| IBIS file generated by GenIBIS.exe Version 3.25
|   am335x_zcz
[IBIS ver]   4.1
[File name]   sprm552c.ibs
[File Rev]   1.1
[Date]   02/05/2016
[Source]   Data created at Texas Instruments
[Notes]   1) Checked with IBISCHK5.0.0 with the following exceptions...
   417 warnings. These warnings can be waived.
   2) Model not valid until this section updated.
   Some pins may contain selectors which are not valid options
   for that particular pin.
   Please refer to the device datasheet for information on picking
   the correct selector model, which depends on various software
   register configurations.
   Some pins are modeled as IO or tri-state for output mode.
[Disclaimer] Please be aware that in the absence of a written agreement,
   Texas Instruments (TI) assumes no liability for: 1) the
   accuracy of the IBIS models provided to your company, 2) the
   proper functioning of these IBIS models in your design or for
   any resulting applications, or, 3) infringement of patents,
   copyrights, or intellectual property rights resulting from
   your use of these IBIS models. TI provides IBIS models as a
   service to our customers and therefore reserves the right to
   limit distribution of the IBIS models.
[Copyright]   Property of Texas Instruments Incorporated. Unauthorised
   reproduction and/or distribution is strictly prohibited. This
   product is protected under copyright law and trade secret law
   as an unpublished work. Created 2016,(C) Copyright 2010,
   Texas Instruments Incorporated., All Rights Reserved. These
   commodities are under the U.S. Government distribution license
   control.As such,they are not to be re-exported without the
   prior approval of the U.S. Department of Commerce.
|   Component am335x_zcz
[Component]   am335x_zce
[Manufacturer]   Texas Instruments.
| Source IO level model revisions
|Model   Revision   Date
|BC1833DV40DCPBFBP18LL_SSDHH   1.1   May 27, 2010
|BC1833DV50BPBFBP18LL_SSDLV   1.0   May 30, 2010
|BC1833DV50BPBFBP18LL_SSDHV   1.1   May 30, 2010
|OQ18SMART1FBPB_SSBHH   1.0   Dec 17, 2008
|BC1833DV40DCPBFBP18LL_SSDLV   1.0   May 27, 2010
|IQ18HYENPB_SSBHH   1.0   May 2, 2008
|BC1833DV50BPBFBP18LL_SSDLH   1.0   May 30, 2010
|BC1833DV40DCPBFBP18LL_SSDHV   1.1   May 27, 2010
|IQ1833DVTCKPBFBP18LL_SSDHH   1.1   May 27, 2010
|IQ18GLFHY_SSBHH   1.0   May 2, 2008
|IHHV1833DVHYP18LL_SSDHH   1.1   May 27, 2010
|BC1833DV50BPBFBP18LL_SSDHH   1.1   May 30, 2010
|BC1833DV40DCPBFBP18LL_SSDLH   1.0   May 27, 2010
|IC1833DVPBFBP18LL_SSDHH   1.1   May 27, 2010
|BCSHTLTCSCDVPBFZ_SSDHV   1.0   May 31, 2010
|BCSHTLTCSCDDVPBFZ_SSDHV   1.0   May 31, 2010
[Package Model] am335x_zce
[Package]
|   typ   min   max
R_pkg   0.22666002591133e-  1.48102e-03   4.40563e-01
L_pkg   3.34766526650246E-009e- 3.63859e-11   7.90050e-09
C_pkg   1.03822401477832E-012e- 3.34415e-13   3.16645e-11
[Pin]   signal_name   model_name
B8   AIN0   NC
A11   AIN1   NC
A8   AIN2   NC
B11   AIN3   NC
C8   AIN4   NC
B12   AIN5   NC
A10   AIN6   NC
A12   AIN7   NC
C13   CAP_VBB_MPU   NC
D6   CAP_VDD_RTC   POWER
B10   CAP_VDD_SRAM_CORE   NC
D13   CAP_VDD_SRAM_MPU   NC
N3   DDR_DQM0   Selector_4
F3   DDR_A0   Selector_4
J1   DDR_VTP   NC
B4   DDR_BA2   Selector_4
H3   DDR_A14   Selector_4
M4   DDR_D11   Selector_11
D2   DDR_A7   Selector_4
G3   DDR_CKE   Selector_4
A3   DDR_BA0   Selector_4
F2   DDR_RASN   Selector_4
P3   DDR_D4   Selector_11
M1   DDR_D13   Selector_11
L1   DDR_DQS1   Selector_1
P1   DDR_D3   Selector_11
F4   DDR_A12   Selector_4
N1   DDR_D15   Selector_11
K2   DDR_D8   Selector_11
R1   DDR_DQS0   Selector_1
L2   DDR_DQSN1   Selector_6
E5   DDR_A4   Selector_4
J2   DDR_A1   Selector_4
G1   DDR_ODT   Selector_4
T1   DDR_D5   Selector_11
A4   DDR_WEN   Selector_4
G4   DDR_A11   Selector_4
E2   DDR_A10   Selector_4
B3   DDR_A3   Selector_4
H2   DDR_CSN0   Selector_4
E3   DDR_A15   Selector_4
G2   DDR_RESETN   Selector_4
C2   DDR_CK   Selector_4
P2   DDR_D2   Selector_11
F1   DDR_CASN   Selector_4
R3   DDR_D7   Selector_11
K3   DDR_DQM1   Selector_4
K1   DDR_D9   Selector_11
A2   DDR_A5   Selector_4
N4   DDR_D0   Selector_11
B2   DDR_A9   Selector_4
M2   DDR_D12   Selector_11
H4   DDR_VREF   NC
N2   DDR_D14   Selector_11
D1   DDR_A2   Selector_4
M3   DDR_D10   Selector_11
R2   DDR_DQSN0   Selector_6
C1   DDR_CKN   Selector_4
T2   DDR_D6   Selector_11
E1   DDR_BA1   Selector_4
H1   DDR_A13   Selector_4
B1   DDR_A6   Selector_4
P4   DDR_D1   Selector_11
C3   DDR_A8   Selector_4
E18   ECAP0_IN_PWM0_OUT   Selector_12
A15   EMU0   Selector_14
D14   EMU1   Selector_14
B5   EXT_WAKEUP   Selector_5
C17   EXTINTN   Selector_7
V17   GPMC_AD15   Selector_15
V15   GPMC_AD8   Selector_15
V12   GPMC_AD2   Selector_15
V10   GPMC_ADVN_ALE   Selector_14
R15   GPMC_WAIT0   Selector_14
U13   GPMC_AD12   Selector_15
T13   GPMC_AD13   Selector_15
U12   GPMC_AD11   Selector_15
V14   GPMC_CSN1   Selector_15
W14   GPMC_AD5   Selector_15
W13   GPMC_AD3   Selector_15
U17   GPMC_CSN3   Selector_15
W8   GPMC_CSN0   Selector_14
T12   GPMC_AD10   Selector_15
U15   GPMC_CSN2   Selector_15
W18   GPMC_WPN   Selector_15
V9   GPMC_AD1   Selector_15
W9   GPMC_OEN_REN   Selector_14
V8   GPMC_BEN0_CLE   Selector_14
W16   GPMC_AD9   Selector_15
V18   GPMC_BEN1   Selector_15
V13   GPMC_AD4   Selector_15
W15   GPMC_AD7   Selector_15
U14   GPMC_AD6   Selector_15
W17   GPMC_AD14   Selector_15
V16   GPMC_CLK   Selector_15
U8   GPMC_WEN   Selector_14
W10   GPMC_AD0   Selector_14
C18   I2C0_SDA   Selector_16
B19   I2C0_SCL   Selector_16
W2   LCD_DATA4   Selector_17
V5   LCD_DATA11   Selector_10
W5   LCD_PCLK   Selector_10
V3   LCD_DATA6   Selector_17
W7   LCD_AC_BIAS_EN   Selector_14
U1   LCD_DATA0   Selector_17
U5   LCD_DATA10   Selector_10
U7   LCD_VSYNC   Selector_14
V2   LCD_DATA3   Selector_17
W3   LCD_DATA5   Selector_17
U6   LCD_DATA13   Selector_17
W4   LCD_DATA9   Selector_10
V7   LCD_DATA15   Selector_14
V6   LCD_DATA12   Selector_17
U3   LCD_DATA7   Selector_10
V1   LCD_DATA2   Selector_17
V4   LCD_DATA8   Selector_10
W6   LCD_DATA14   Selector_15
T7   LCD_HSYNC   Selector_14
U2   LCD_DATA1   Selector_17
R19   MDC   Selector_10
P17   MDIO   Selector_10
L18   MII1_TXD0   Selector_10
J18   MII1_CRS   Selector_10
N18   MII1_TXD2   Selector_10
J19   MII1_COL   Selector_10
N19   MII1_TX_CLK   Selector_10
M17   MII1_TXD3   Selector_10
M18   MII1_TXD1   Selector_10
N16   MII1_RXD2   Selector_10
M19   MII1_RX_CLK   Selector_10
P18   MII1_RXD0   Selector_10
K19   MII1_RX_ER   Selector_10
K17   MII1_TX_EN   Selector_10
P19   MII1_RXD1   Selector_10
N17   MII1_RXD3   Selector_10
L19   MII1_RX_DV   Selector_10
G17   MMC0_CMD   Selector_10
H17   MMC0_DAT1   Selector_10
H18   MMC0_DAT2   Selector_10
G19   MMC0_CLK   Selector_10
G18   MMC0_DAT0   Selector_10
H19   MMC0_DAT3   Selector_10
C7   PMIC_POWER_EN   Selector_2
E15   PWRONRSTN   Selector_3
B6   RESERVED   NC
K18   RMII1_REF_CLK   Selector_10
B7   RTC_PWRONRSTN   Model_172
A6   RTC_XTALIN   NC
A5   RTC_XTALOUT   NC
A7   RTC_KALDO_ENN   NC
A18   SPI0_SCLK   Selector_14
B16   SPI0_CS1   Selector_14
B18   SPI0_D0   Selector_14
A17   SPI0_CS0   Selector_14
B17   SPI0_D1   Selector_14
B14   TCK   Selector_8
B13   TDI   Selector_19
A14   TDO   Selector_13
C14   TMS   Selector_18
A13   TRSTN   Selector_19
E19   UART0_RXD   Selector_12
F17   UART0_TXD   Selector_12
F18   UART0_RTSN   Selector_12
F19   UART0_CTSN   Selector_12
D18   UART1_RXD   Selector_12
D19   UART1_RTSN   Selector_12
C19   UART1_TXD   Selector_12
E17   UART1_CTSN   Selector_12
T18   USB0_CE   NC
U18   USB0_DM   NC
T19   USB0_VBUS   NC
V19   USB0_ID   NC
G16   USB0_DRVVBUS   Selector_12
U19   USB0_DP   NC
F11   VDD_CORE   POWER
F9   VDD_CORE   POWER
G11   VDD_CORE   POWER
G9   VDD_CORE   POWER
H12   VDD_CORE   POWER
H13   VDD_CORE   POWER
H7   VDD_CORE   POWER
H8   VDD_CORE   POWER
J12   VDD_CORE   POWER
J13   VDD_CORE   POWER
J7   VDD_CORE   POWER
J8   VDD_CORE   POWER
K15   VDD_CORE   POWER
K16   VDD_CORE   POWER
L12   VDD_CORE   POWER
L13   VDD_CORE   POWER
L7   VDD_CORE   POWER
L8   VDD_CORE   POWER
M12   VDD_CORE   POWER
M13   VDD_CORE   POWER
M7   VDD_CORE   POWER
M8   VDD_CORE   POWER
N11   VDD_CORE   POWER
N9   VDD_CORE   POWER
P11   VDD_CORE   POWER
P9   VDD_CORE   POWER
D7   VDDA_ADC   POWER
R17   VDDA1P8V_USB0   POWER
R18   VDDA3P3V_USB0   POWER
G5   VDDS_DDR   POWER
H5   VDDS_DDR   POWER
H6   VDDS_DDR   POWER
K4   VDDS_DDR   POWER
K5   VDDS_DDR   POWER
M5   VDDS_DDR   POWER
M6   VDDS_DDR   POWER
N5   VDDS_DDR   POWER
U10   VDDS_OSC   POWER
C6   VDDS_RTC   POWER
C5   VDDS_PLL_DDR   POWER
D12   VDDS   POWER
F16   VDDS   POWER
M16   VDDS   POWER
T14   VDDS   POWER
T6   VDDS   POWER
T8   VDDS_PLL_CORE_LCD   POWER
C12   VDDS_SRAM_MPU_BB   POWER
H16   VDDS_PLL_MPU   POWER
C10   VDDS_SRAM_CORE_BG   POWER
R11   VDDSHV1   POWER
R12   VDDSHV1   POWER
R13   VDDSHV1   POWER
R8   VDDSHV1   POWER
R9   VDDSHV1   POWER
G15   VDDSHV4   POWER
H14   VDDSHV4   POWER
H15   VDDSHV4   POWER
M14   VDDSHV5   POWER
M15   VDDSHV5   POWER
N15   VDDSHV5   POWER
E11   VDDSHV6   POWER
E12   VDDSHV6   POWER
E13   VDDSHV6   POWER
F14   VDDSHV6   POWER
P6   VDDSHV6   POWER
R7   VDDSHV6   POWER
R5   VPP   POWER
B9   VREFN   NC
A9   VREFP   NC
V11   VSS_OSC   GND
A1   VSS   GND
A19   VSS   GND
D10   VSS   GND
E10   VSS   GND
E7   VSS   GND
E8   VSS   GND
E9   VSS   GND
F12   VSS   GND
F13   VSS   GND
F6   VSS   GND
F7   VSS   GND
F8   VSS   GND
G12   VSS   GND
G8   VSS   GND
H10   VSS   GND
H11   VSS   GND
H9   VSS   GND
J11   VSS   GND
J14   VSS   GND
J15   VSS   GND
J5   VSS   GND
J6   VSS   GND
J9   VSS   GND
K11   VSS   GND
K12   VSS   GND
K8   VSS   GND
K9   VSS   GND
L11   VSS   GND
L14   VSS   GND
L15   VSS   GND
L5   VSS   GND
L6   VSS   GND
L9   VSS   GND
M10   VSS   GND
M11   VSS   GND
M9   VSS   GND
N12   VSS   GND
N8   VSS   GND
P12   VSS   GND
P13   VSS   GND
P14   VSS   GND
P7   VSS   GND
P8   VSS   GND
R10   VSS   GND
T10   VSS   GND
W1   VSS   GND
W19   VSS   GND
P16   VSSA_USB   GND
D8   VSSA_ADC   GND
A16   WARMRSTN   Selector_9
C15   XDMA_EVENT_INTR0   Selector_16
B15   XDMA_EVENT_INTR1   Selector_16
W11   XTALIN   NC
W12   XTALOUT   NC
[Diff Pin] inv_pin  vdiff  tdelay_typ
|Differential signal data for cell BCSHTLTCSCDDVPBFZ_SSDHV
|DDR_DQS1   DDR_DQSN1
L1   L2   200m   NA
|DDR_DQS0   DDR_DQSN0
R1   R2   200m   NA
|   Usage INPUT#1.35/1.5V/1.8V#X#X#BCSHTLTCSCDDVPBFZ_SSDHV.PADP
|   OUTPUT#1.35/1.5V/1.8V#X#X#BCSHTLTCSCDDVPBFZ_SSDHV.TX_P
|   Base model BCSHTLTCSCDDVPBFZ_SSDHV
[Model Selector] Selector_1
Model_1000 INPUT,1.5V,FULLTERM, 1.00*RExt,IND,5%,DIFF_VREF_FULLTERM_8MA_5PER_1P5
Model_1001 INPUT,1.5V,Half Thevenin, 1.60*RExt,IND,5%,DIFF_VREF_HALFTERM_5MA_5PER
Model_1002 INPUT,1.5V,FULLTERM, 0.88*RExt,IND,5%,DIFF_VREF_FULLTERM_9MA_5PER_1P5
Model_1003 INPUT,1.35V,Half Thevenin, 0.67*RExt,IND,10%,DIFF_VREF_HALFTERM_12MA_1
Model_1004 INPUT,1.35V,Pull-up/down off,IND,10%,DIFF_VREF_NOTERM_PUPD_OFF_10PER_1
Model_1005 INPUT,1.35V,FULLTERM, 1.60*RExt,IND,10%,DIFF_VREF_FULLTERM_5MA_10PER_1
Model_1006 INPUT,1.35V,Half Thevenin, 1.60*RExt,IND,10%,DIFF_VREF_HALFTERM_5MA_10
Model_1007 INPUT,1.35V,Pull-up,IND,10%,DIFF_VREF_NOTERM_PU_ON_10PER_1P35
Model_1008 INPUT,1.35V,FULLTERM, 0.88*RExt,IND,10%,DIFF_VREF_FULLTERM_9MA_10PER_1
Model_1009 INPUT,1.35V,FULLTERM, 1.14*RExt,IND,10%,DIFF_VREF_FULLTERM_7MA_10PER_1
Model_1010 INPUT,1.35V,Half Thevenin, 0.88*RExt,IND,10%,DIFF_VREF_HALFTERM_9MA_10
Model_1011 INPUT,1.35V,FULLTERM, 1.33*RExt,IND,10%,DIFF_VREF_FULLTERM_6MA_10PER_1
Model_1012 INPUT,1.35V,Half Thevenin, 1.14*RExt,IND,10%,DIFF_VREF_HALFTERM_7MA_10
Model_1013 INPUT,1.35V,Half Thevenin, 1.33*RExt,IND,10%,DIFF_VREF_HALFTERM_6MA_10
Model_1014 INPUT,1.35V,FULLTERM, 0.73*RExt,IND,10%,DIFF_VREF_FULLTERM_11MA_10PER_
Model_1015 INPUT,1.35V,FULLTERM, 0.80*RExt,IND,10%,DIFF_VREF_FULLTERM_10MA_10PER_
Model_1016 INPUT,1.35V,Half Thevenin, 0.73*RExt,IND,10%,DIFF_VREF_HALFTERM_11MA_1
Model_1017 INPUT,1.35V,FULLTERM, 1.00*RExt,IND,10%,DIFF_VREF_FULLTERM_8MA_10PER_1
Model_1018 INPUT,1.35V,Half Thevenin, 0.80*RExt,IND,10%,DIFF_VREF_HALFTERM_10MA_1
Model_1019 INPUT,1.35V,Pull-down,IND,10%,DIFF_VREF_NOTERM_PD_ON_10PER_1P35
Model_1020 INPUT,1.35V,Half Thevenin, 1.00*RExt,IND,10%,DIFF_VREF_HALFTERM_8MA_10
Model_1021 INPUT,1.35V,FULLTERM, 0.67*RExt,IND,10%,DIFF_VREF_FULLTERM_12MA_10PER_
Model_1022 INPUT,1.35V,Half Thevenin, 0.67*RExt,IND,5%,DIFF_VREF_HALFTERM_12MA_5P
Model_1023 INPUT,1.35V,Pull-up/down off,IND,5%,DIFF_VREF_NOTERM_PUPD_OFF_5PER_1P3
Model_1024 INPUT,1.35V,FULLTERM, 1.60*RExt,IND,5%,DIFF_VREF_FULLTERM_5MA_5PER_1P3
Model_1025 INPUT,1.35V,Half Thevenin, 1.60*RExt,IND,5%,DIFF_VREF_HALFTERM_5MA_5PE
Model_1026 INPUT,1.35V,Pull-up,IND,5%,DIFF_VREF_NOTERM_PU_ON_5PER_1P35
Model_1027 INPUT,1.35V,FULLTERM, 0.88*RExt,IND,5%,DIFF_VREF_FULLTERM_9MA_5PER_1P3
Model_1028 INPUT,1.35V,FULLTERM, 1.14*RExt,IND,5%,DIFF_VREF_FULLTERM_7MA_5PER_1P3
Model_1029 INPUT,1.35V,Half Thevenin, 0.88*RExt,IND,5%,DIFF_VREF_HALFTERM_9MA_5PE
Model_1030 INPUT,1.35V,FULLTERM, 1.33*RExt,IND,5%,DIFF_VREF_FULLTERM_6MA_5PER_1P3
Model_1031 INPUT,1.35V,Half Thevenin, 1.14*RExt,IND,5%,DIFF_VREF_HALFTERM_7MA_5PE
Model_1032 INPUT,1.35V,Half Thevenin, 1.33*RExt,IND,5%,DIFF_VREF_HALFTERM_6MA_5PE
Model_1033 INPUT,1.35V,FULLTERM, 0.73*RExt,IND,5%,DIFF_VREF_FULLTERM_11MA_5PER_1P
Model_1034 INPUT,1.35V,FULLTERM, 0.80*RExt,IND,5%,DIFF_VREF_FULLTERM_10MA_5PER_1P
Model_1035 INPUT,1.35V,Half Thevenin, 0.73*RExt,IND,5%,DIFF_VREF_HALFTERM_11MA_5P
Model_1036 INPUT,1.35V,FULLTERM, 1.00*RExt,IND,5%,DIFF_VREF_FULLTERM_8MA_5PER_1P3
Model_1037 INPUT,1.35V,Half Thevenin, 0.80*RExt,IND,5%,DIFF_VREF_HALFTERM_10MA_5P
Model_1038 INPUT,1.35V,Pull-down,IND,5%,DIFF_VREF_NOTERM_PD_ON_5PER_1P35
Model_1039 INPUT,1.35V,Half Thevenin, 1.00*RExt,IND,5%,DIFF_VREF_HALFTERM_8MA_5PE
Model_1040 INPUT,1.35V,FULLTERM, 0.67*RExt,IND,5%,DIFF_VREF_FULLTERM_12MA_5PER_1P
Model_537 3-STATE,1.8V,ODT off,slowest, 1.00*RExt,IND,10%,SR11_8MA_PADP_10PER_1P
Model_538 3-STATE,1.8V,ODT off,slowest, 1.60*RExt,IND,10%,SR11_5MA_PADP_10PER_1P
Model_539 3-STATE,1.8V,ODT off,fast, 1.14*RExt,IND,10%,SR10_7MA_PADP_10PER_1P8
Model_540 3-STATE,1.8V,ODT off,fast, 1.33*RExt,IND,10%,SR10_6MA_PADP_10PER_1P8
Model_541 3-STATE,1.8V,ODT off,slowest, 0.88*RExt,IND,10%,SR11_9MA_PADP_10PER_1P
Model_542 3-STATE,1.8V,ODT off,fast, 0.73*RExt,IND,10%,SR10_11MA_PADP_10PER_1P8
Model_543 3-STATE,1.8V,ODT off,slowest, 0.67*RExt,IND,10%,SR11_12MA_PADP_10PER_1
Model_544 3-STATE,1.8V,ODT off,slowest, 1.14*RExt,IND,10%,SR11_7MA_PADP_10PER_1P
Model_545 3-STATE,1.8V,ODT off,fast, 0.80*RExt,IND,10%,SR10_10MA_PADP_10PER_1P8
Model_546 3-STATE,1.8V,ODT off,slowest, 1.33*RExt,IND,10%,SR11_6MA_PADP_10PER_1P
Model_547 3-STATE,1.8V,ODT off,fast, 1.00*RExt,IND,10%,SR10_8MA_PADP_10PER_1P8
Model_548 3-STATE,1.8V,ODT off,fast, 1.60*RExt,IND,10%,SR10_5MA_PADP_10PER_1P8
Model_549 3-STATE,1.8V,ODT off,slowest, 0.73*RExt,IND,10%,SR11_11MA_PADP_10PER_1
Model_550 3-STATE,1.8V,ODT off,slowest, 0.80*RExt,IND,10%,SR11_10MA_PADP_10PER_1
Model_551 3-STATE,1.8V,ODT off,fast, 0.88*RExt,IND,10%,SR10_9MA_PADP_10PER_1P8
Model_552 3-STATE,1.8V,ODT off,fast, 0.67*RExt,IND,10%,SR10_12MA_PADP_10PER_1P8
Model_553 3-STATE,1.8V,ODT off,slowest, 1.00*RExt,IND,5%,SR11_8MA_PADP_5PER_1P8
Model_554 3-STATE,1.8V,ODT off,slowest, 1.60*RExt,IND,5%,SR11_5MA_PADP_5PER_1P8
Model_555 3-STATE,1.8V,ODT off,fast, 1.14*RExt,IND,5%,SR10_7MA_PADP_5PER_1P8
Model_556 3-STATE,1.8V,ODT off,fast, 1.33*RExt,IND,5%,SR10_6MA_PADP_5PER_1P8
Model_557 3-STATE,1.8V,ODT off,slowest, 0.88*RExt,IND,5%,SR11_9MA_PADP_5PER_1P8
Model_558 3-STATE,1.8V,ODT off,fast, 0.73*RExt,IND,5%,SR10_11MA_PADP_5PER_1P8
Model_559 3-STATE,1.8V,ODT off,slowest, 0.67*RExt,IND,5%,SR11_12MA_PADP_5PER_1P8
Model_560 3-STATE,1.8V,ODT off,slowest, 1.14*RExt,IND,5%,SR11_7MA_PADP_5PER_1P8
Model_561 3-STATE,1.8V,ODT off,fast, 0.80*RExt,IND,5%,SR10_10MA_PADP_5PER_1P8
Model_562 3-STATE,1.8V,ODT off,slowest, 1.33*RExt,IND,5%,SR11_6MA_PADP_5PER_1P8
Model_563 3-STATE,1.8V,ODT off,fast, 1.00*RExt,IND,5%,SR10_8MA_PADP_5PER_1P8
Model_564 3-STATE,1.8V,ODT off,fast, 1.60*RExt,IND,5%,SR10_5MA_PADP_5PER_1P8
Model_565 3-STATE,1.8V,ODT off,slowest, 0.73*RExt,IND,5%,SR11_11MA_PADP_5PER_1P8
Model_566 3-STATE,1.8V,ODT off,slowest, 0.80*RExt,IND,5%,SR11_10MA_PADP_5PER_1P8
Model_567 3-STATE,1.8V,ODT off,fast, 0.88*RExt,IND,5%,SR10_9MA_PADP_5PER_1P8
Model_568 3-STATE,1.8V,ODT off,fast, 0.67*RExt,IND,5%,SR10_12MA_PADP_5PER_1P8
Model_569 3-STATE,1.5V,ODT off,slowest, 1.00*RExt,IND,10%,SR11_8MA_PADP_10PER_1P
Model_570 3-STATE,1.5V,ODT off,slowest, 1.60*RExt,IND,10%,SR11_5MA_PADP_10PER_1P
Model_571 3-STATE,1.5V,ODT off,fast, 1.14*RExt,IND,10%,SR10_7MA_PADP_10PER_1P5
Model_572 3-STATE,1.5V,ODT off,fast, 1.33*RExt,IND,10%,SR10_6MA_PADP_10PER_1P5
Model_573 3-STATE,1.5V,ODT off,slowest, 0.88*RExt,IND,10%,SR11_9MA_PADP_10PER_1P
Model_574 3-STATE,1.5V,ODT off,fast, 0.73*RExt,IND,10%,SR10_11MA_PADP_10PER_1P5
Model_575 3-STATE,1.5V,ODT off,slowest, 0.67*RExt,IND,10%,SR11_12MA_PADP_10PER_1
Model_576 3-STATE,1.5V,ODT off,slowest, 1.14*RExt,IND,10%,SR11_7MA_PADP_10PER_1P
Model_577 3-STATE,1.5V,ODT off,fast, 0.80*RExt,IND,10%,SR10_10MA_PADP_10PER_1P5
Model_578 3-STATE,1.5V,ODT off,slowest, 1.33*RExt,IND,10%,SR11_6MA_PADP_10PER_1P
Model_579 3-STATE,1.5V,ODT off,fast, 1.00*RExt,IND,10%,SR10_8MA_PADP_10PER_1P5
Model_580 3-STATE,1.5V,ODT off,fast, 1.60*RExt,IND,10%,SR10_5MA_PADP_10PER_1P5
Model_581 3-STATE,1.5V,ODT off,slowest, 0.73*RExt,IND,10%,SR11_11MA_PADP_10PER_1
Model_582 3-STATE,1.5V,ODT off,slowest, 0.80*RExt,IND,10%,SR11_10MA_PADP_10PER_1
Model_583 3-STATE,1.5V,ODT off,fast, 0.88*RExt,IND,10%,SR10_9MA_PADP_10PER_1P5
Model_584 3-STATE,1.5V,ODT off,fast, 0.67*RExt,IND,10%,SR10_12MA_PADP_10PER_1P5
Model_585 3-STATE,1.5V,ODT off,slowest, 1.00*RExt,IND,5%,SR11_8MA_PADP_5PER_1P5
Model_586 3-STATE,1.5V,ODT off,slowest, 1.60*RExt,IND,5%,SR11_5MA_PADP_5PER_1P5
Model_587 3-STATE,1.5V,ODT off,fast, 1.14*RExt,IND,5%,SR10_7MA_PADP_5PER_1P5
Model_588 3-STATE,1.5V,ODT off,fast, 1.33*RExt,IND,5%,SR10_6MA_PADP_5PER_1P5
Model_589 3-STATE,1.5V,ODT off,slowest, 0.88*RExt,IND,5%,SR11_9MA_PADP_5PER_1P5
Model_590 3-STATE,1.5V,ODT off,fast, 0.73*RExt,IND,5%,SR10_11MA_PADP_5PER_1P5
Model_591 3-STATE,1.5V,ODT off,slowest, 0.67*RExt,IND,5%,SR11_12MA_PADP_5PER_1P5
Model_592 3-STATE,1.5V,ODT off,slowest, 1.14*RExt,IND,5%,SR11_7MA_PADP_5PER_1P5
Model_593 3-STATE,1.5V,ODT off,fast, 0.80*RExt,IND,5%,SR10_10MA_PADP_5PER_1P5
Model_594 3-STATE,1.5V,ODT off,slowest, 1.33*RExt,IND,5%,SR11_6MA_PADP_5PER_1P5
Model_595 3-STATE,1.5V,ODT off,fast, 1.00*RExt,IND,5%,SR10_8MA_PADP_5PER_1P5
Model_596 3-STATE,1.5V,ODT off,fast, 1.60*RExt,IND,5%,SR10_5MA_PADP_5PER_1P5
Model_597 3-STATE,1.5V,ODT off,slowest, 0.73*RExt,IND,5%,SR11_11MA_PADP_5PER_1P5
Model_598 3-STATE,1.5V,ODT off,slowest, 0.80*RExt,IND,5%,SR11_10MA_PADP_5PER_1P5
Model_599 3-STATE,1.5V,ODT off,fast, 0.88*RExt,IND,5%,SR10_9MA_PADP_5PER_1P5
Model_600 3-STATE,1.5V,ODT off,fast, 0.67*RExt,IND,5%,SR10_12MA_PADP_5PER_1P5
Model_601 3-STATE,1.8V,ODT off,slow, 0.67*RExt,IND,10%,SR01_12MA_PADP_10PER_1P8
Model_602 3-STATE,1.8V,ODT off,fastest, 1.60*RExt,IND,10%,SR00_5MA_PADP_10PER_1P
Model_603 3-STATE,1.8V,ODT off,fastest, 0.88*RExt,IND,10%,SR00_9MA_PADP_10PER_1P
Model_604 3-STATE,1.8V,ODT off,slow, 1.60*RExt,IND,10%,SR01_5MA_PADP_10PER_1P8
Model_605 3-STATE,1.8V,ODT off,fastest, 1.14*RExt,IND,10%,SR00_7MA_PADP_10PER_1P
Model_606 3-STATE,1.8V,ODT off,fastest, 1.33*RExt,IND,10%,SR00_6MA_PADP_10PER_1P
Model_607 3-STATE,1.8V,ODT off,slow, 0.88*RExt,IND,10%,SR01_9MA_PADP_10PER_1P8
Model_608 3-STATE,1.8V,ODT off,fastest, 0.73*RExt,IND,10%,SR00_11MA_PADP_10PER_1
Model_609 3-STATE,1.8V,ODT off,slow, 1.14*RExt,IND,10%,SR01_7MA_PADP_10PER_1P8
Model_610 3-STATE,1.8V,ODT off,fastest, 0.80*RExt,IND,10%,SR00_10MA_PADP_10PER_1
Model_611 3-STATE,1.8V,ODT off,slow, 1.33*RExt,IND,10%,SR01_6MA_PADP_10PER_1P8
Model_612 3-STATE,1.8V,ODT off,fastest, 1.00*RExt,IND,10%,SR00_8MA_PADP_10PER_1P
Model_613 3-STATE,1.8V,ODT off,slow, 0.73*RExt,IND,10%,SR01_11MA_PADP_10PER_1P8
Model_614 3-STATE,1.8V,ODT off,slow, 0.80*RExt,IND,10%,SR01_10MA_PADP_10PER_1P8
Model_615 3-STATE,1.8V,ODT off,fastest, 0.67*RExt,IND,10%,SR00_12MA_PADP_10PER_1
Model_616 3-STATE,1.8V,ODT off,slow, 1.00*RExt,IND,10%,SR01_8MA_PADP_10PER_1P8
Model_617 3-STATE,1.8V,ODT off,slow, 0.67*RExt,IND,5%,SR01_12MA_PADP_5PER_1P8
Model_618 3-STATE,1.8V,ODT off,fastest, 1.60*RExt,IND,5%,SR00_5MA_PADP_5PER_1P8
Model_619 3-STATE,1.8V,ODT off,fastest, 0.88*RExt,IND,5%,SR00_9MA_PADP_5PER_1P8
Model_620 3-STATE,1.8V,ODT off,slow, 1.60*RExt,IND,5%,SR01_5MA_PADP_5PER_1P8
Model_621 3-STATE,1.8V,ODT off,fastest, 1.14*RExt,IND,5%,SR00_7MA_PADP_5PER_1P8
Model_622 3-STATE,1.8V,ODT off,fastest, 1.33*RExt,IND,5%,SR00_6MA_PADP_5PER_1P8
Model_623 3-STATE,1.8V,ODT off,slow, 0.88*RExt,IND,5%,SR01_9MA_PADP_5PER_1P8
Model_624 3-STATE,1.8V,ODT off,fastest, 0.73*RExt,IND,5%,SR00_11MA_PADP_5PER_1P8
Model_625 3-STATE,1.8V,ODT off,slow, 1.14*RExt,IND,5%,SR01_7MA_PADP_5PER_1P8
Model_626 3-STATE,1.8V,ODT off,fastest, 0.80*RExt,IND,5%,SR00_10MA_PADP_5PER_1P8
Model_627 3-STATE,1.8V,ODT off,slow, 1.33*RExt,IND,5%,SR01_6MA_PADP_5PER_1P8
Model_628 3-STATE,1.8V,ODT off,fastest, 1.00*RExt,IND,5%,SR00_8MA_PADP_5PER_1P8
Model_629 3-STATE,1.8V,ODT off,slow, 0.73*RExt,IND,5%,SR01_11MA_PADP_5PER_1P8
Model_630 3-STATE,1.8V,ODT off,slow, 0.80*RExt,IND,5%,SR01_10MA_PADP_5PER_1P8
Model_631 3-STATE,1.8V,ODT off,fastest, 0.67*RExt,IND,5%,SR00_12MA_PADP_5PER_1P8
Model_632 3-STATE,1.8V,ODT off,slow, 1.00*RExt,IND,5%,SR01_8MA_PADP_5PER_1P8
Model_633 3-STATE,1.5V,ODT off,slow, 0.67*RExt,IND,10%,SR01_12MA_PADP_10PER_1P5
Model_634 3-STATE,1.5V,ODT off,fastest, 1.60*RExt,IND,10%,SR00_5MA_PADP_10PER_1P
Model_635 3-STATE,1.5V,ODT off,fastest, 0.88*RExt,IND,10%,SR00_9MA_PADP_10PER_1P
Model_636 3-STATE,1.5V,ODT off,slow, 1.60*RExt,IND,10%,SR01_5MA_PADP_10PER_1P5
Model_637 3-STATE,1.5V,ODT off,fastest, 1.14*RExt,IND,10%,SR00_7MA_PADP_10PER_1P
Model_638 3-STATE,1.5V,ODT off,fastest, 1.33*RExt,IND,10%,SR00_6MA_PADP_10PER_1P
Model_639 3-STATE,1.5V,ODT off,slow, 0.88*RExt,IND,10%,SR01_9MA_PADP_10PER_1P5
Model_640 3-STATE,1.5V,ODT off,fastest, 0.73*RExt,IND,10%,SR00_11MA_PADP_10PER_1
Model_641 3-STATE,1.5V,ODT off,slow, 1.14*RExt,IND,10%,SR01_7MA_PADP_10PER_1P5
Model_642 3-STATE,1.5V,ODT off,fastest, 0.80*RExt,IND,10%,SR00_10MA_PADP_10PER_1
Model_643 3-STATE,1.5V,ODT off,slow, 1.33*RExt,IND,10%,SR01_6MA_PADP_10PER_1P5
Model_644 3-STATE,1.5V,ODT off,fastest, 1.00*RExt,IND,10%,SR00_8MA_PADP_10PER_1P
Model_645 3-STATE,1.5V,ODT off,slow, 0.73*RExt,IND,10%,SR01_11MA_PADP_10PER_1P5
Model_646 3-STATE,1.5V,ODT off,slow, 0.80*RExt,IND,10%,SR01_10MA_PADP_10PER_1P5
Model_647 3-STATE,1.5V,ODT off,fastest, 0.67*RExt,IND,10%,SR00_12MA_PADP_10PER_1
Model_648 3-STATE,1.5V,ODT off,slow, 1.00*RExt,IND,10%,SR01_8MA_PADP_10PER_1P5
Model_649 3-STATE,1.5V,ODT off,slow, 0.67*RExt,IND,5%,SR01_12MA_PADP_5PER_1P5
Model_650 3-STATE,1.5V,ODT off,fastest, 1.60*RExt,IND,5%,SR00_5MA_PADP_5PER_1P5
Model_651 3-STATE,1.5V,ODT off,fastest, 0.88*RExt,IND,5%,SR00_9MA_PADP_5PER_1P5
Model_652 3-STATE,1.5V,ODT off,slow, 1.60*RExt,IND,5%,SR01_5MA_PADP_5PER_1P5
Model_653 3-STATE,1.5V,ODT off,fastest, 1.14*RExt,IND,5%,SR00_7MA_PADP_5PER_1P5
Model_654 3-STATE,1.5V,ODT off,fastest, 1.33*RExt,IND,5%,SR00_6MA_PADP_5PER_1P5
Model_655 3-STATE,1.5V,ODT off,slow, 0.88*RExt,IND,5%,SR01_9MA_PADP_5PER_1P5
Model_656 3-STATE,1.5V,ODT off,fastest, 0.73*RExt,IND,5%,SR00_11MA_PADP_5PER_1P5
Model_657 3-STATE,1.5V,ODT off,slow, 1.14*RExt,IND,5%,SR01_7MA_PADP_5PER_1P5
Model_658 3-STATE,1.5V,ODT off,fastest, 0.80*RExt,IND,5%,SR00_10MA_PADP_5PER_1P5
Model_659 3-STATE,1.5V,ODT off,slow, 1.33*RExt,IND,5%,SR01_6MA_PADP_5PER_1P5
Model_660 3-STATE,1.5V,ODT off,fastest, 1.00*RExt,IND,5%,SR00_8MA_PADP_5PER_1P5
Model_661 3-STATE,1.5V,ODT off,slow, 0.73*RExt,IND,5%,SR01_11MA_PADP_5PER_1P5
Model_662 3-STATE,1.5V,ODT off,slow, 0.80*RExt,IND,5%,SR01_10MA_PADP_5PER_1P5
Model_663 3-STATE,1.5V,ODT off,fastest, 0.67*RExt,IND,5%,SR00_12MA_PADP_5PER_1P5
Model_664 3-STATE,1.5V,ODT off,slow, 1.00*RExt,IND,5%,SR01_8MA_PADP_5PER_1P5
Model_665 3-STATE,1.35V,ODT off,slowest, 0.67*RExt,IND,10%,SR11_12MA_PADP_10PER_
Model_666 3-STATE,1.35V,ODT off,fast, 1.60*RExt,IND,10%,SR10_5MA_PADP_10PER_1P35
Model_667 3-STATE,1.35V,ODT off,fast, 0.88*RExt,IND,10%,SR10_9MA_PADP_10PER_1P35
Model_668 3-STATE,1.35V,ODT off,slow, 1.60*RExt,IND,10%,SR01_5MA_PADP_10PER_1P35
Model_669 3-STATE,1.35V,ODT off,slowest, 1.60*RExt,IND,10%,SR11_5MA_PADP_10PER_1
Model_670 3-STATE,1.35V,ODT off,fastest, 1.14*RExt,IND,10%,SR00_7MA_PADP_10PER_1
Model_671 3-STATE,1.35V,ODT off,slow, 0.88*RExt,IND,10%,SR01_9MA_PADP_10PER_1P35
Model_672 3-STATE,1.35V,ODT off,fastest, 0.73*RExt,IND,10%,SR00_11MA_PADP_10PER_
Model_673 3-STATE,1.35V,ODT off,fastest, 0.80*RExt,IND,10%,SR00_10MA_PADP_10PER_
Model_674 3-STATE,1.35V,ODT off,fast, 0.73*RExt,IND,10%,SR10_11MA_PADP_10PER_1P3
Model_675 3-STATE,1.35V,ODT off,slowest, 1.14*RExt,IND,10%,SR11_7MA_PADP_10PER_1
Model_676 3-STATE,1.35V,ODT off,fast, 1.00*RExt,IND,10%,SR10_8MA_PADP_10PER_1P35
Model_677 3-STATE,1.35V,ODT off,slow, 0.73*RExt,IND,10%,SR01_11MA_PADP_10PER_1P3
Model_678 3-STATE,1.35V,ODT off,slow, 1.00*RExt,IND,10%,SR01_8MA_PADP_10PER_1P35
Model_679 3-STATE,1.35V,ODT off,fast, 0.67*RExt,IND,10%,SR10_12MA_PADP_10PER_1P3
Model_680 3-STATE,1.35V,ODT off,slowest, 1.00*RExt,IND,10%,SR11_8MA_PADP_10PER_1
Model_681 3-STATE,1.35V,ODT off,slow, 0.67*RExt,IND,10%,SR01_12MA_PADP_10PER_1P3
Model_682 3-STATE,1.35V,ODT off,fastest, 1.60*RExt,IND,10%,SR00_5MA_PADP_10PER_1
Model_683 3-STATE,1.35V,ODT off,fastest, 0.88*RExt,IND,10%,SR00_9MA_PADP_10PER_1
Model_684 3-STATE,1.35V,ODT off,fastest, 1.33*RExt,IND,10%,SR00_6MA_PADP_10PER_1
Model_685 3-STATE,1.35V,ODT off,fast, 1.14*RExt,IND,10%,SR10_7MA_PADP_10PER_1P35
Model_686 3-STATE,1.35V,ODT off,fast, 1.33*RExt,IND,10%,SR10_6MA_PADP_10PER_1P35
Model_687 3-STATE,1.35V,ODT off,slow, 1.14*RExt,IND,10%,SR01_7MA_PADP_10PER_1P35
Model_688 3-STATE,1.35V,ODT off,slowest, 0.88*RExt,IND,10%,SR11_9MA_PADP_10PER_1
Model_689 3-STATE,1.35V,ODT off,slow, 1.33*RExt,IND,10%,SR01_6MA_PADP_10PER_1P35
Model_690 3-STATE,1.35V,ODT off,fastest, 1.00*RExt,IND,10%,SR00_8MA_PADP_10PER_1
Model_691 3-STATE,1.35V,ODT off,fast, 0.80*RExt,IND,10%,SR10_10MA_PADP_10PER_1P3
Model_692 3-STATE,1.35V,ODT off,slowest, 1.33*RExt,IND,10%,SR11_6MA_PADP_10PER_1
Model_693 3-STATE,1.35V,ODT off,slow, 0.80*RExt,IND,10%,SR01_10MA_PADP_10PER_1P3
Model_694 3-STATE,1.35V,ODT off,fastest, 0.67*RExt,IND,10%,SR00_12MA_PADP_10PER_
Model_695 3-STATE,1.35V,ODT off,slowest, 0.73*RExt,IND,10%,SR11_11MA_PADP_10PER_
Model_696 3-STATE,1.35V,ODT off,slowest, 0.80*RExt,IND,10%,SR11_10MA_PADP_10PER_
Model_697 3-STATE,1.35V,ODT off,slowest, 0.67*RExt,IND,5%,SR11_12MA_PADP_5PER_1P
Model_698 3-STATE,1.35V,ODT off,fast, 1.60*RExt,IND,5%,SR10_5MA_PADP_5PER_1P35
Model_699 3-STATE,1.35V,ODT off,fast, 0.88*RExt,IND,5%,SR10_9MA_PADP_5PER_1P35
Model_700 3-STATE,1.35V,ODT off,slow, 1.60*RExt,IND,5%,SR01_5MA_PADP_5PER_1P35
Model_701 3-STATE,1.35V,ODT off,slowest, 1.60*RExt,IND,5%,SR11_5MA_PADP_5PER_1P3
Model_702 3-STATE,1.35V,ODT off,fastest, 1.14*RExt,IND,5%,SR00_7MA_PADP_5PER_1P3
Model_703 3-STATE,1.35V,ODT off,slow, 0.88*RExt,IND,5%,SR01_9MA_PADP_5PER_1P35
Model_704 3-STATE,1.35V,ODT off,fastest, 0.73*RExt,IND,5%,SR00_11MA_PADP_5PER_1P
Model_705 3-STATE,1.35V,ODT off,fastest, 0.80*RExt,IND,5%,SR00_10MA_PADP_5PER_1P
Model_706 3-STATE,1.35V,ODT off,fast, 0.73*RExt,IND,5%,SR10_11MA_PADP_5PER_1P35
Model_707 3-STATE,1.35V,ODT off,slowest, 1.14*RExt,IND,5%,SR11_7MA_PADP_5PER_1P3
Model_708 3-STATE,1.35V,ODT off,fast, 1.00*RExt,IND,5%,SR10_8MA_PADP_5PER_1P35
Model_709 3-STATE,1.35V,ODT off,slow, 0.73*RExt,IND,5%,SR01_11MA_PADP_5PER_1P35
Model_710 3-STATE,1.35V,ODT off,slow, 1.00*RExt,IND,5%,SR01_8MA_PADP_5PER_1P35
Model_711 3-STATE,1.35V,ODT off,fast, 0.67*RExt,IND,5%,SR10_12MA_PADP_5PER_1P35
Model_712 3-STATE,1.35V,ODT off,slowest, 1.00*RExt,IND,5%,SR11_8MA_PADP_5PER_1P3
Model_713 3-STATE,1.35V,ODT off,slow, 0.67*RExt,IND,5%,SR01_12MA_PADP_5PER_1P35
Model_714 3-STATE,1.35V,ODT off,fastest, 1.60*RExt,IND,5%,SR00_5MA_PADP_5PER_1P3
Model_715 3-STATE,1.35V,ODT off,fastest, 0.88*RExt,IND,5%,SR00_9MA_PADP_5PER_1P3
Model_716 3-STATE,1.35V,ODT off,fastest, 1.33*RExt,IND,5%,SR00_6MA_PADP_5PER_1P3
Model_717 3-STATE,1.35V,ODT off,fast, 1.14*RExt,IND,5%,SR10_7MA_PADP_5PER_1P35
Model_718 3-STATE,1.35V,ODT off,fast, 1.33*RExt,IND,5%,SR10_6MA_PADP_5PER_1P35
Model_719 3-STATE,1.35V,ODT off,slow, 1.14*RExt,IND,5%,SR01_7MA_PADP_5PER_1P35
Model_720 3-STATE,1.35V,ODT off,slowest, 0.88*RExt,IND,5%,SR11_9MA_PADP_5PER_1P3
Model_721 3-STATE,1.35V,ODT off,slow, 1.33*RExt,IND,5%,SR01_6MA_PADP_5PER_1P35
Model_722 3-STATE,1.35V,ODT off,fastest, 1.00*RExt,IND,5%,SR00_8MA_PADP_5PER_1P3
Model_723 3-STATE,1.35V,ODT off,fast, 0.80*RExt,IND,5%,SR10_10MA_PADP_5PER_1P35
Model_724 3-STATE,1.35V,ODT off,slowest, 1.33*RExt,IND,5%,SR11_6MA_PADP_5PER_1P3
Model_725 3-STATE,1.35V,ODT off,slow, 0.80*RExt,IND,5%,SR01_10MA_PADP_5PER_1P35
Model_726 3-STATE,1.35V,ODT off,fastest, 0.67*RExt,IND,5%,SR00_12MA_PADP_5PER_1P
Model_727 3-STATE,1.35V,ODT off,slowest, 0.73*RExt,IND,5%,SR11_11MA_PADP_5PER_1P
Model_728 3-STATE,1.35V,ODT off,slowest, 0.80*RExt,IND,5%,SR11_10MA_PADP_5PER_1P
Model_921 INPUT,1.8V,Half Thevenin, 0.67*RExt,IND,10%,DIFF_VREF_HALFTERM_12MA_10
Model_922 INPUT,1.8V,Pull-up/down off,IND,10%,DIFF_VREF_NOTERM_PUPD_OFF_10PER_1P
Model_923 INPUT,1.8V,Pull-down,IND,10%,DIFF_LVCMOS_PD_ON_10PER_1P8
Model_924 INPUT,1.8V,FULLTERM, 1.60*RExt,IND,10%,DIFF_VREF_FULLTERM_5MA_10PER_1P
Model_925 INPUT,1.8V,Half Thevenin, 1.60*RExt,IND,10%,DIFF_VREF_HALFTERM_5MA_10P
Model_926 INPUT,1.8V,Pull-up,IND,10%,DIFF_VREF_NOTERM_PU_ON_10PER_1P8
Model_927 INPUT,1.8V,FULLTERM, 0.88*RExt,IND,10%,DIFF_VREF_FULLTERM_9MA_10PER_1P
Model_928 INPUT,1.8V,FULLTERM, 1.14*RExt,IND,10%,DIFF_VREF_FULLTERM_7MA_10PER_1P
Model_929 INPUT,1.8V,Half Thevenin, 0.88*RExt,IND,10%,DIFF_VREF_HALFTERM_9MA_10P
Model_930 INPUT,1.8V,FULLTERM, 1.33*RExt,IND,10%,DIFF_VREF_FULLTERM_6MA_10PER_1P
Model_931 INPUT,1.8V,Half Thevenin, 1.14*RExt,IND,10%,DIFF_VREF_HALFTERM_7MA_10P
Model_932 INPUT,1.8V,Half Thevenin, 1.33*RExt,IND,10%,DIFF_VREF_HALFTERM_6MA_10P
Model_933 INPUT,1.8V,FULLTERM, 0.73*RExt,IND,10%,DIFF_VREF_FULLTERM_11MA_10PER_1
Model_934 INPUT,1.8V,Pull-up/down off,IND,10%,DIFF_LVCMOS_PUPD_OFF_10PER_1P8
Model_935 INPUT,1.8V,FULLTERM, 0.80*RExt,IND,10%,DIFF_VREF_FULLTERM_10MA_10PER_1
Model_936 INPUT,1.8V,Half Thevenin, 0.73*RExt,IND,10%,DIFF_VREF_HALFTERM_11MA_10
Model_937 INPUT,1.8V,FULLTERM, 1.00*RExt,IND,10%,DIFF_VREF_FULLTERM_8MA_10PER_1P
Model_938 INPUT,1.8V,Half Thevenin, 0.80*RExt,IND,10%,DIFF_VREF_HALFTERM_10MA_10
Model_939 INPUT,1.8V,Pull-down,IND,10%,DIFF_VREF_NOTERM_PD_ON_10PER_1P8
Model_940 INPUT,1.8V,Half Thevenin, 1.00*RExt,IND,10%,DIFF_VREF_HALFTERM_8MA_10P
Model_941 INPUT,1.8V,Pull-up,IND,10%,DIFF_LVCMOS_PU_ON_10PER_1P8
Model_942 INPUT,1.8V,FULLTERM, 0.67*RExt,IND,10%,DIFF_VREF_FULLTERM_12MA_10PER_1
Model_943 INPUT,1.8V,Half Thevenin, 0.67*RExt,IND,5%,DIFF_VREF_HALFTERM_12MA_5PE
Model_944 INPUT,1.8V,Pull-up/down off,IND,5%,DIFF_VREF_NOTERM_PUPD_OFF_5PER_1P8
Model_945 INPUT,1.8V,Pull-down,IND,5%,DIFF_LVCMOS_PD_ON_5PER_1P8
Model_946 INPUT,1.8V,FULLTERM, 1.60*RExt,IND,5%,DIFF_VREF_FULLTERM_5MA_5PER_1P8
Model_947 INPUT,1.8V,Half Thevenin, 1.60*RExt,IND,5%,DIFF_VREF_HALFTERM_5MA_5PER
Model_948 INPUT,1.8V,Pull-up,IND,5%,DIFF_VREF_NOTERM_PU_ON_5PER_1P8
Model_949 INPUT,1.8V,FULLTERM, 0.88*RExt,IND,5%,DIFF_VREF_FULLTERM_9MA_5PER_1P8
Model_950 INPUT,1.8V,FULLTERM, 1.14*RExt,IND,5%,DIFF_VREF_FULLTERM_7MA_5PER_1P8
Model_951 INPUT,1.8V,Half Thevenin, 0.88*RExt,IND,5%,DIFF_VREF_HALFTERM_9MA_5PER
Model_952 INPUT,1.8V,FULLTERM, 1.33*RExt,IND,5%,DIFF_VREF_FULLTERM_6MA_5PER_1P8
Model_953 INPUT,1.8V,Half Thevenin, 1.14*RExt,IND,5%,DIFF_VREF_HALFTERM_7MA_5PER
Model_954 INPUT,1.8V,Half Thevenin, 1.33*RExt,IND,5%,DIFF_VREF_HALFTERM_6MA_5PER
Model_955 INPUT,1.8V,FULLTERM, 0.73*RExt,IND,5%,DIFF_VREF_FULLTERM_11MA_5PER_1P8
Model_956 INPUT,1.8V,Pull-up/down off,IND,5%,DIFF_LVCMOS_PUPD_OFF_5PER_1P8
Model_957 INPUT,1.8V,FULLTERM, 0.80*RExt,IND,5%,DIFF_VREF_FULLTERM_10MA_5PER_1P8
Model_958 INPUT,1.8V,Half Thevenin, 0.73*RExt,IND,5%,DIFF_VREF_HALFTERM_11MA_5PE
Model_959 INPUT,1.8V,FULLTERM, 1.00*RExt,IND,5%,DIFF_VREF_FULLTERM_8MA_5PER_1P8
Model_960 INPUT,1.8V,Half Thevenin, 0.80*RExt,IND,5%,DIFF_VREF_HALFTERM_10MA_5PE
Model_961 INPUT,1.8V,Pull-down,IND,5%,DIFF_VREF_NOTERM_PD_ON_5PER_1P8
Model_962 INPUT,1.8V,Half Thevenin, 1.00*RExt,IND,5%,DIFF_VREF_HALFTERM_8MA_5PER
Model_963 INPUT,1.8V,Pull-up,IND,5%,DIFF_LVCMOS_PU_ON_5PER_1P8
Model_964 INPUT,1.8V,FULLTERM, 0.67*RExt,IND,5%,DIFF_VREF_FULLTERM_12MA_5PER_1P8
Model_965 INPUT,1.5V,FULLTERM, 1.14*RExt,IND,10%,DIFF_VREF_FULLTERM_7MA_10PER_1P
Model_966 INPUT,1.5V,FULLTERM, 1.33*RExt,IND,10%,DIFF_VREF_FULLTERM_6MA_10PER_1P
Model_967 INPUT,1.5V,Half Thevenin, 0.67*RExt,IND,10%,DIFF_VREF_HALFTERM_12MA_10
Model_968 INPUT,1.5V,FULLTERM, 1.60*RExt,IND,10%,DIFF_VREF_FULLTERM_5MA_10PER_1P
Model_969 INPUT,1.5V,Pull-up,IND,10%,DIFF_VREF_NOTERM_PU_ON_10PER_1P5
Model_970 INPUT,1.5V,Half Thevenin, 0.73*RExt,IND,10%,DIFF_VREF_HALFTERM_11MA_10
Model_971 INPUT,1.5V,Half Thevenin, 0.80*RExt,IND,10%,DIFF_VREF_HALFTERM_10MA_10
Model_972 INPUT,1.5V,Half Thevenin, 1.00*RExt,IND,10%,DIFF_VREF_HALFTERM_8MA_10P
Model_973 INPUT,1.5V,FULLTERM, 0.67*RExt,IND,10%,DIFF_VREF_FULLTERM_12MA_10PER_1
Model_974 INPUT,1.5V,Half Thevenin, 0.88*RExt,IND,10%,DIFF_VREF_HALFTERM_9MA_10P
Model_975 INPUT,1.5V,Pull-up/down off,IND,10%,DIFF_VREF_NOTERM_PUPD_OFF_10PER_1P
Model_976 INPUT,1.5V,Half Thevenin, 1.14*RExt,IND,10%,DIFF_VREF_HALFTERM_7MA_10P
Model_977 INPUT,1.5V,Half Thevenin, 1.33*RExt,IND,10%,DIFF_VREF_HALFTERM_6MA_10P
Model_978 INPUT,1.5V,FULLTERM, 0.73*RExt,IND,10%,DIFF_VREF_FULLTERM_11MA_10PER_1
Model_979 INPUT,1.5V,FULLTERM, 0.80*RExt,IND,10%,DIFF_VREF_FULLTERM_10MA_10PER_1
Model_980 INPUT,1.5V,Pull-down,IND,10%,DIFF_VREF_NOTERM_PD_ON_10PER_1P5
Model_981 INPUT,1.5V,FULLTERM, 1.00*RExt,IND,10%,DIFF_VREF_FULLTERM_8MA_10PER_1P
Model_982 INPUT,1.5V,Half Thevenin, 1.60*RExt,IND,10%,DIFF_VREF_HALFTERM_5MA_10P
Model_983 INPUT,1.5V,FULLTERM, 0.88*RExt,IND,10%,DIFF_VREF_FULLTERM_9MA_10PER_1P
Model_984 INPUT,1.5V,FULLTERM, 1.14*RExt,IND,5%,DIFF_VREF_FULLTERM_7MA_5PER_1P5
Model_985 INPUT,1.5V,FULLTERM, 1.33*RExt,IND,5%,DIFF_VREF_FULLTERM_6MA_5PER_1P5
Model_986 INPUT,1.5V,Half Thevenin, 0.67*RExt,IND,5%,DIFF_VREF_HALFTERM_12MA_5PE
Model_987 INPUT,1.5V,FULLTERM, 1.60*RExt,IND,5%,DIFF_VREF_FULLTERM_5MA_5PER_1P5
Model_988 INPUT,1.5V,Pull-up,IND,5%,DIFF_VREF_NOTERM_PU_ON_5PER_1P5
Model_989 INPUT,1.5V,Half Thevenin, 0.73*RExt,IND,5%,DIFF_VREF_HALFTERM_11MA_5PE
Model_990 INPUT,1.5V,Half Thevenin, 0.80*RExt,IND,5%,DIFF_VREF_HALFTERM_10MA_5PE
Model_991 INPUT,1.5V,Half Thevenin, 1.00*RExt,IND,5%,DIFF_VREF_HALFTERM_8MA_5PER
Model_992 INPUT,1.5V,FULLTERM, 0.67*RExt,IND,5%,DIFF_VREF_FULLTERM_12MA_5PER_1P5
Model_993 INPUT,1.5V,Half Thevenin, 0.88*RExt,IND,5%,DIFF_VREF_HALFTERM_9MA_5PER
Model_994 INPUT,1.5V,Pull-up/down off,IND,5%,DIFF_VREF_NOTERM_PUPD_OFF_5PER_1P5
Model_995 INPUT,1.5V,Half Thevenin, 1.14*RExt,IND,5%,DIFF_VREF_HALFTERM_7MA_5PER
Model_996 INPUT,1.5V,Half Thevenin, 1.33*RExt,IND,5%,DIFF_VREF_HALFTERM_6MA_5PER
Model_997 INPUT,1.5V,FULLTERM, 0.73*RExt,IND,5%,DIFF_VREF_FULLTERM_11MA_5PER_1P5
Model_998 INPUT,1.5V,FULLTERM, 0.80*RExt,IND,5%,DIFF_VREF_FULLTERM_10MA_5PER_1P5
Model_999 INPUT,1.5V,Pull-down,IND,5%,DIFF_VREF_NOTERM_PD_ON_5PER_1P5
|   Usage OUTPUT#1.8V#X#X#OQ18SMART1FBPB_SSBHH.PAD
|   Base model OQ18SMART1FBPB_SSBHH
[Model Selector] Selector_2
Model_49 3-STATE,1.8V,Pull-up,S00, L01,SBHH_HS00L01_PU1_1P8
Model_50 3-STATE,1.8V,Pull-down,S01, L11,SBHH_HS01L11_PD1_1P8
Model_51 3-STATE,1.8V,Pull-down,S01, L10,SBHH_HS01L10_PD1_1P8
Model_52 3-STATE,1.8V,Pull-up,S11, L11,SBHH_HS11L11_PU1_1P8
Model_53 3-STATE,1.8V,Pull-down,S00, L11,SBHH_HS00L11_PD1_1P8
Model_54 3-STATE,1.8V,Pull-up/down off,S11, L10,HH_HS11L10_PUPD0_1P8
Model_55 3-STATE,1.8V,Pull-up,S10, L11,SBHH_HS10L11_PU1_1P8
Model_56 3-STATE,1.8V,Pull-down,S00, L10,SBHH_HS00L10_PD1_1P8
Model_57 3-STATE,1.8V,Pull-up/down off,S10, L10,HH_HS10L10_PUPD0_1P8
Model_58 3-STATE,1.8V,Pull-up,S10, L10,SBHH_HS10L10_PU1_1P8
Model_59 3-STATE,1.8V,Pull-up/down off,S11, L00,HH_HS11L00_PUPD0_1P8
Model_60 3-STATE,1.8V,Pull-down,S00, L01,SBHH_HS00L01_PD1_1P8
Model_61 3-STATE,1.8V,Pull-up/down off,S10, L01,HH_HS10L01_PUPD0_1P8
Model_62 3-STATE,1.8V,Pull-up/down off,S10, L00,HH_HS10L00_PUPD0_1P8
Model_63 3-STATE,1.8V,Pull-down,S11, L11,SBHH_HS11L11_PD1_1P8
Model_64 3-STATE,1.8V,Pull-up,S01, L11,SBHH_HS01L11_PU1_1P8
Model_65 3-STATE,1.8V,Pull-up/down off,S01, L10,HH_HS01L10_PUPD0_1P8
Model_66 3-STATE,1.8V,Pull-up,S01, L10,SBHH_HS01L10_PU1_1P8
Model_67 3-STATE,1.8V,Pull-down,S10, L01,SBHH_HS10L01_PD1_1P8
Model_68 3-STATE,1.8V,Pull-up/down off,S01, L01,HH_HS01L01_PUPD0_1P8
Model_69 3-STATE,1.8V,Pull-up/down off,S01, L00,HH_HS01L00_PUPD0_1P8
Model_70 3-STATE,1.8V,Pull-down,S10, L00,SBHH_HS10L00_PD1_1P8
Model_71 3-STATE,1.8V,Pull-up/down off,S00, L01,HH_HS00L01_PUPD0_1P8
Model_72 3-STATE,1.8V,Pull-up/down off,S00, L00,HH_HS00L00_PUPD0_1P8
Model_73 3-STATE,1.8V,Pull-up,S00, L00,SBHH_HS00L00_PU1_1P8
Model_74 3-STATE,1.8V,Pull-up,S11, L10,SBHH_HS11L10_PU1_1P8
Model_75 3-STATE,1.8V,Pull-up/down off,S11, L11,HH_HS11L11_PUPD0_1P8
Model_76 3-STATE,1.8V,Pull-up/down off,S10, L11,HH_HS10L11_PUPD0_1P8
Model_77 3-STATE,1.8V,Pull-down,S01, L01,SBHH_HS01L01_PD1_1P8
Model_78 3-STATE,1.8V,Pull-up,S11, L01,SBHH_HS11L01_PU1_1P8
Model_79 3-STATE,1.8V,Pull-up/down off,S11, L01,HH_HS11L01_PUPD0_1P8
Model_80 3-STATE,1.8V,Pull-down,S01, L00,SBHH_HS01L00_PD1_1P8
Model_81 3-STATE,1.8V,Pull-up,S11, L00,SBHH_HS11L00_PU1_1P8
Model_82 3-STATE,1.8V,Pull-up,S10, L01,SBHH_HS10L01_PU1_1P8
Model_83 3-STATE,1.8V,Pull-down,S00, L00,SBHH_HS00L00_PD1_1P8
Model_84 3-STATE,1.8V,Pull-up,S10, L00,SBHH_HS10L00_PU1_1P8
Model_85 3-STATE,1.8V,Pull-down,S11, L10,SBHH_HS11L10_PD1_1P8
Model_86 3-STATE,1.8V,Pull-down,S10, L11,SBHH_HS10L11_PD1_1P8
Model_87 3-STATE,1.8V,Pull-up/down off,S01, L11,HH_HS01L11_PUPD0_1P8
Model_88 3-STATE,1.8V,Pull-down,S10, L10,SBHH_HS10L10_PD1_1P8
Model_89 3-STATE,1.8V,Pull-down,S11, L01,SBHH_HS11L01_PD1_1P8
Model_90 3-STATE,1.8V,Pull-up,S00, L11,SBHH_HS00L11_PU1_1P8
Model_91 3-STATE,1.8V,Pull-up/down off,S00, L11,HH_HS00L11_PUPD0_1P8
Model_92 3-STATE,1.8V,Pull-down,S11, L00,SBHH_HS11L00_PD1_1P8
Model_93 3-STATE,1.8V,Pull-up/down off,S00, L10,HH_HS00L10_PUPD0_1P8
Model_94 3-STATE,1.8V,Pull-up,S01, L01,SBHH_HS01L01_PU1_1P8
Model_95 3-STATE,1.8V,Pull-up,S00, L10,SBHH_HS00L10_PU1_1P8
Model_96 3-STATE,1.8V,Pull-up,S01, L00,SBHH_HS01L00_PU1_1P8
|   Usage INPUT#1.8V/3.3V#X#X#IHHV1833DVHYP18LL_SSDHH.PAD
|   Base model IHHV1833DVHYP18LL_SSDHH
[Model Selector] Selector_3
Model_173 INPUT,1.8V,NORMAL,IND,5%,IHHV_NORAML_5P_1P8
Model_174 INPUT,3.3V,NORMAL,IND,5%,IHHV_NORAML_5P_3P3
Model_175 INPUT,1.8V,NORMAL,IND,10%,IHHV_NORAML_10P_1P8
Model_176 INPUT,3.3V,NORMAL,IND,10%,IHHV_NORAML_10P_3P3
|   Usage OUTPUT#1.35/1.5V/1.8V#X#X#BCSHTLTCSCDVPBFZ_SSDHV.PAD
|   Base model BCSHTLTCSCDVPBFZ_SSDHV
[Model Selector] Selector_4
Model_225 3-STATE,1.8V,ODT off,slowest, 1.00*RExt,IND,10%,SR11_8MA_10PER_1P8
Model_226 3-STATE,1.8V,ODT off,slowest, 1.60*RExt,IND,10%,SR11_5MA_10PER_1P8
Model_227 3-STATE,1.8V,ODT off,fast, 1.14*RExt,IND,10%,SR10_7MA_10PER_1P8
Model_228 3-STATE,1.8V,ODT off,fast, 1.33*RExt,IND,10%,SR10_6MA_10PER_1P8
Model_229 3-STATE,1.8V,ODT off,slowest, 0.88*RExt,IND,10%,SR11_9MA_10PER_1P8
Model_230 3-STATE,1.8V,ODT off,fast, 0.73*RExt,IND,10%,SR10_11MA_10PER_1P8
Model_231 3-STATE,1.8V,ODT off,slowest, 0.67*RExt,IND,10%,SR11_12MA_10PER_1P8
Model_232 3-STATE,1.8V,ODT off,slowest, 1.14*RExt,IND,10%,SR11_7MA_10PER_1P8
Model_233 3-STATE,1.8V,ODT off,fast, 0.80*RExt,IND,10%,SR10_10MA_10PER_1P8
Model_234 3-STATE,1.8V,ODT off,slowest, 1.33*RExt,IND,10%,SR11_6MA_10PER_1P8
Model_235 3-STATE,1.8V,ODT off,fast, 1.00*RExt,IND,10%,SR10_8MA_10PER_1P8
Model_236 3-STATE,1.8V,ODT off,fast, 1.60*RExt,IND,10%,SR10_5MA_10PER_1P8
Model_237 3-STATE,1.8V,ODT off,slowest, 0.73*RExt,IND,10%,SR11_11MA_10PER_1P8
Model_238 3-STATE,1.8V,ODT off,slowest, 0.80*RExt,IND,10%,SR11_10MA_10PER_1P8
Model_239 3-STATE,1.8V,ODT off,fast, 0.88*RExt,IND,10%,SR10_9MA_10PER_1P8
Model_240 3-STATE,1.8V,ODT off,fast, 0.67*RExt,IND,10%,SR10_12MA_10PER_1P8
Model_241 3-STATE,1.8V,ODT off,slowest, 1.00*RExt,IND,5%,SR11_8MA_5PER_1P8
Model_242 3-STATE,1.8V,ODT off,slowest, 1.60*RExt,IND,5%,SR11_5MA_5PER_1P8
Model_243 3-STATE,1.8V,ODT off,fast, 1.14*RExt,IND,5%,SR10_7MA_5PER_1P8
Model_244 3-STATE,1.8V,ODT off,fast, 1.33*RExt,IND,5%,SR10_6MA_5PER_1P8
Model_245 3-STATE,1.8V,ODT off,slowest, 0.88*RExt,IND,5%,SR11_9MA_5PER_1P8
Model_246 3-STATE,1.8V,ODT off,fast, 0.73*RExt,IND,5%,SR10_11MA_5PER_1P8
Model_247 3-STATE,1.8V,ODT off,slowest, 0.67*RExt,IND,5%,SR11_12MA_5PER_1P8
Model_248 3-STATE,1.8V,ODT off,slowest, 1.14*RExt,IND,5%,SR11_7MA_5PER_1P8
Model_249 3-STATE,1.8V,ODT off,fast, 0.80*RExt,IND,5%,SR10_10MA_5PER_1P8
Model_250 3-STATE,1.8V,ODT off,slowest, 1.33*RExt,IND,5%,SR11_6MA_5PER_1P8
Model_251 3-STATE,1.8V,ODT off,fast, 1.00*RExt,IND,5%,SR10_8MA_5PER_1P8
Model_252 3-STATE,1.8V,ODT off,fast, 1.60*RExt,IND,5%,SR10_5MA_5PER_1P8
Model_253 3-STATE,1.8V,ODT off,slowest, 0.73*RExt,IND,5%,SR11_11MA_5PER_1P8
Model_254 3-STATE,1.8V,ODT off,slowest, 0.80*RExt,IND,5%,SR11_10MA_5PER_1P8
Model_255 3-STATE,1.8V,ODT off,fast, 0.88*RExt,IND,5%,SR10_9MA_5PER_1P8
Model_256 3-STATE,1.8V,ODT off,fast, 0.67*RExt,IND,5%,SR10_12MA_5PER_1P8
Model_257 3-STATE,1.5V,ODT off,slowest, 1.00*RExt,IND,10%,SR11_8MA_10PER_1P5
Model_258 3-STATE,1.5V,ODT off,slowest, 1.60*RExt,IND,10%,SR11_5MA_10PER_1P5
Model_259 3-STATE,1.5V,ODT off,fast, 1.14*RExt,IND,10%,SR10_7MA_10PER_1P5
Model_260 3-STATE,1.5V,ODT off,fast, 1.33*RExt,IND,10%,SR10_6MA_10PER_1P5
Model_261 3-STATE,1.5V,ODT off,slowest, 0.88*RExt,IND,10%,SR11_9MA_10PER_1P5
Model_262 3-STATE,1.5V,ODT off,fast, 0.73*RExt,IND,10%,SR10_11MA_10PER_1P5
Model_263 3-STATE,1.5V,ODT off,slowest, 0.67*RExt,IND,10%,SR11_12MA_10PER_1P5
Model_264 3-STATE,1.5V,ODT off,slowest, 1.14*RExt,IND,10%,SR11_7MA_10PER_1P5
Model_265 3-STATE,1.5V,ODT off,fast, 0.80*RExt,IND,10%,SR10_10MA_10PER_1P5
Model_266 3-STATE,1.5V,ODT off,slowest, 1.33*RExt,IND,10%,SR11_6MA_10PER_1P5
Model_267 3-STATE,1.5V,ODT off,fast, 1.00*RExt,IND,10%,SR10_8MA_10PER_1P5
Model_268 3-STATE,1.5V,ODT off,fast, 1.60*RExt,IND,10%,SR10_5MA_10PER_1P5
Model_269 3-STATE,1.5V,ODT off,slowest, 0.73*RExt,IND,10%,SR11_11MA_10PER_1P5
Model_270 3-STATE,1.5V,ODT off,slowest, 0.80*RExt,IND,10%,SR11_10MA_10PER_1P5
Model_271 3-STATE,1.5V,ODT off,fast, 0.88*RExt,IND,10%,SR10_9MA_10PER_1P5
Model_272 3-STATE,1.5V,ODT off,fast, 0.67*RExt,IND,10%,SR10_12MA_10PER_1P5
Model_273 3-STATE,1.5V,ODT off,slowest, 1.00*RExt,IND,5%,SR11_8MA_5PER_1P5
Model_274 3-STATE,1.5V,ODT off,slowest, 1.60*RExt,IND,5%,SR11_5MA_5PER_1P5
Model_275 3-STATE,1.5V,ODT off,fast, 1.14*RExt,IND,5%,SR10_7MA_5PER_1P5
Model_276 3-STATE,1.5V,ODT off,fast, 1.33*RExt,IND,5%,SR10_6MA_5PER_1P5
Model_277 3-STATE,1.5V,ODT off,slowest, 0.88*RExt,IND,5%,SR11_9MA_5PER_1P5
Model_278 3-STATE,1.5V,ODT off,fast, 0.73*RExt,IND,5%,SR10_11MA_5PER_1P5
Model_279 3-STATE,1.5V,ODT off,slowest, 0.67*RExt,IND,5%,SR11_12MA_5PER_1P5
Model_280 3-STATE,1.5V,ODT off,slowest, 1.14*RExt,IND,5%,SR11_7MA_5PER_1P5
Model_281 3-STATE,1.5V,ODT off,fast, 0.80*RExt,IND,5%,SR10_10MA_5PER_1P5
Model_282 3-STATE,1.5V,ODT off,slowest, 1.33*RExt,IND,5%,SR11_6MA_5PER_1P5
Model_283 3-STATE,1.5V,ODT off,fast, 1.00*RExt,IND,5%,SR10_8MA_5PER_1P5
Model_284 3-STATE,1.5V,ODT off,fast, 1.60*RExt,IND,5%,SR10_5MA_5PER_1P5
Model_285 3-STATE,1.5V,ODT off,slowest, 0.73*RExt,IND,5%,SR11_11MA_5PER_1P5
Model_286 3-STATE,1.5V,ODT off,slowest, 0.80*RExt,IND,5%,SR11_10MA_5PER_1P5
Model_287 3-STATE,1.5V,ODT off,fast, 0.88*RExt,IND,5%,SR10_9MA_5PER_1P5
Model_288 3-STATE,1.5V,ODT off,fast, 0.67*RExt,IND,5%,SR10_12MA_5PER_1P5
Model_289 3-STATE,1.8V,ODT off,slow, 0.67*RExt,IND,10%,SR01_12MA_10PER_1P8
Model_290 3-STATE,1.8V,ODT off,fastest, 1.60*RExt,IND,10%,SR00_5MA_10PER_1P8
Model_291 3-STATE,1.8V,ODT off,fastest, 0.88*RExt,IND,10%,SR00_9MA_10PER_1P8
Model_292 3-STATE,1.8V,ODT off,slow, 1.60*RExt,IND,10%,SR01_5MA_10PER_1P8
Model_293 3-STATE,1.8V,ODT off,fastest, 1.14*RExt,IND,10%,SR00_7MA_10PER_1P8
Model_294 3-STATE,1.8V,ODT off,fastest, 1.33*RExt,IND,10%,SR00_6MA_10PER_1P8
Model_295 3-STATE,1.8V,ODT off,slow, 0.88*RExt,IND,10%,SR01_9MA_10PER_1P8
Model_296 3-STATE,1.8V,ODT off,fastest, 0.73*RExt,IND,10%,SR00_11MA_10PER_1P8
Model_297 3-STATE,1.8V,ODT off,slow, 1.14*RExt,IND,10%,SR01_7MA_10PER_1P8
Model_298 3-STATE,1.8V,ODT off,fastest, 0.80*RExt,IND,10%,SR00_10MA_10PER_1P8
Model_299 3-STATE,1.8V,ODT off,slow, 1.33*RExt,IND,10%,SR01_6MA_10PER_1P8
Model_300 3-STATE,1.8V,ODT off,fastest, 1.00*RExt,IND,10%,SR00_8MA_10PER_1P8
Model_301 3-STATE,1.8V,ODT off,slow, 0.73*RExt,IND,10%,SR01_11MA_10PER_1P8
Model_302 3-STATE,1.8V,ODT off,slow, 0.80*RExt,IND,10%,SR01_10MA_10PER_1P8
Model_303 3-STATE,1.8V,ODT off,fastest, 0.67*RExt,IND,10%,SR00_12MA_10PER_1P8
Model_304 3-STATE,1.8V,ODT off,slow, 1.00*RExt,IND,10%,SR01_8MA_10PER_1P8
Model_305 3-STATE,1.8V,ODT off,slow, 0.67*RExt,IND,5%,SR01_12MA_5PER_1P8
Model_306 3-STATE,1.8V,ODT off,fastest, 1.60*RExt,IND,5%,SR00_5MA_5PER_1P8
Model_307 3-STATE,1.8V,ODT off,fastest, 0.88*RExt,IND,5%,SR00_9MA_5PER_1P8
Model_308 3-STATE,1.8V,ODT off,slow, 1.60*RExt,IND,5%,SR01_5MA_5PER_1P8
Model_309 3-STATE,1.8V,ODT off,fastest, 1.14*RExt,IND,5%,SR00_7MA_5PER_1P8
Model_310 3-STATE,1.8V,ODT off,fastest, 1.33*RExt,IND,5%,SR00_6MA_5PER_1P8
Model_311 3-STATE,1.8V,ODT off,slow, 0.88*RExt,IND,5%,SR01_9MA_5PER_1P8
Model_312 3-STATE,1.8V,ODT off,fastest, 0.73*RExt,IND,5%,SR00_11MA_5PER_1P8
Model_313 3-STATE,1.8V,ODT off,slow, 1.14*RExt,IND,5%,SR01_7MA_5PER_1P8
Model_314 3-STATE,1.8V,ODT off,fastest, 0.80*RExt,IND,5%,SR00_10MA_5PER_1P8
Model_315 3-STATE,1.8V,ODT off,slow, 1.33*RExt,IND,5%,SR01_6MA_5PER_1P8
Model_316 3-STATE,1.8V,ODT off,fastest, 1.00*RExt,IND,5%,SR00_8MA_5PER_1P8
Model_317 3-STATE,1.8V,ODT off,slow, 0.73*RExt,IND,5%,SR01_11MA_5PER_1P8
Model_318 3-STATE,1.8V,ODT off,slow, 0.80*RExt,IND,5%,SR01_10MA_5PER_1P8
Model_319 3-STATE,1.8V,ODT off,fastest, 0.67*RExt,IND,5%,SR00_12MA_5PER_1P8
Model_320 3-STATE,1.8V,ODT off,slow, 1.00*RExt,IND,5%,SR01_8MA_5PER_1P8
Model_321 3-STATE,1.5V,ODT off,slow, 0.67*RExt,IND,10%,SR01_12MA_10PER_1P5
Model_322 3-STATE,1.5V,ODT off,fastest, 1.60*RExt,IND,10%,SR00_5MA_10PER_1P5
Model_323 3-STATE,1.5V,ODT off,fastest, 0.88*RExt,IND,10%,SR00_9MA_10PER_1P5
Model_324 3-STATE,1.5V,ODT off,slow, 1.60*RExt,IND,10%,SR01_5MA_10PER_1P5
Model_325 3-STATE,1.5V,ODT off,fastest, 1.14*RExt,IND,10%,SR00_7MA_10PER_1P5
Model_326 3-STATE,1.5V,ODT off,fastest, 1.33*RExt,IND,10%,SR00_6MA_10PER_1P5
Model_327 3-STATE,1.5V,ODT off,slow, 0.88*RExt,IND,10%,SR01_9MA_10PER_1P5
Model_328 3-STATE,1.5V,ODT off,fastest, 0.73*RExt,IND,10%,SR00_11MA_10PER_1P5
Model_329 3-STATE,1.5V,ODT off,slow, 1.14*RExt,IND,10%,SR01_7MA_10PER_1P5
Model_330 3-STATE,1.5V,ODT off,fastest, 0.80*RExt,IND,10%,SR00_10MA_10PER_1P5
Model_331 3-STATE,1.5V,ODT off,slow, 1.33*RExt,IND,10%,SR01_6MA_10PER_1P5
Model_332 3-STATE,1.5V,ODT off,fastest, 1.00*RExt,IND,10%,SR00_8MA_10PER_1P5
Model_333 3-STATE,1.5V,ODT off,slow, 0.73*RExt,IND,10%,SR01_11MA_10PER_1P5
Model_334 3-STATE,1.5V,ODT off,slow, 0.80*RExt,IND,10%,SR01_10MA_10PER_1P5
Model_335 3-STATE,1.5V,ODT off,fastest, 0.67*RExt,IND,10%,SR00_12MA_10PER_1P5
Model_336 3-STATE,1.5V,ODT off,slow, 1.00*RExt,IND,10%,SR01_8MA_10PER_1P5
Model_337 3-STATE,1.5V,ODT off,slow, 0.67*RExt,IND,5%,SR01_12MA_5PER_1P5
Model_338 3-STATE,1.5V,ODT off,fastest, 1.60*RExt,IND,5%,SR00_5MA_5PER_1P5
Model_339 3-STATE,1.5V,ODT off,fastest, 0.88*RExt,IND,5%,SR00_9MA_5PER_1P5
Model_340 3-STATE,1.5V,ODT off,slow, 1.60*RExt,IND,5%,SR01_5MA_5PER_1P5
Model_341 3-STATE,1.5V,ODT off,fastest, 1.14*RExt,IND,5%,SR00_7MA_5PER_1P5
Model_342 3-STATE,1.5V,ODT off,fastest, 1.33*RExt,IND,5%,SR00_6MA_5PER_1P5
Model_343 3-STATE,1.5V,ODT off,slow, 0.88*RExt,IND,5%,SR01_9MA_5PER_1P5
Model_344 3-STATE,1.5V,ODT off,fastest, 0.73*RExt,IND,5%,SR00_11MA_5PER_1P5
Model_345 3-STATE,1.5V,ODT off,slow, 1.14*RExt,IND,5%,SR01_7MA_5PER_1P5
Model_346 3-STATE,1.5V,ODT off,fastest, 0.80*RExt,IND,5%,SR00_10MA_5PER_1P5
Model_347 3-STATE,1.5V,ODT off,slow, 1.33*RExt,IND,5%,SR01_6MA_5PER_1P5
Model_348 3-STATE,1.5V,ODT off,fastest, 1.00*RExt,IND,5%,SR00_8MA_5PER_1P5
Model_349 3-STATE,1.5V,ODT off,slow, 0.73*RExt,IND,5%,SR01_11MA_5PER_1P5
Model_350 3-STATE,1.5V,ODT off,slow, 0.80*RExt,IND,5%,SR01_10MA_5PER_1P5
Model_351 3-STATE,1.5V,ODT off,fastest, 0.67*RExt,IND,5%,SR00_12MA_5PER_1P5
Model_352 3-STATE,1.5V,ODT off,slow, 1.00*RExt,IND,5%,SR01_8MA_5PER_1P5
Model_353 3-STATE,1.35V,ODT off,slowest, 0.67*RExt,IND,10%,SR11_12MA_10PER_1P35
Model_354 3-STATE,1.35V,ODT off,fast, 1.60*RExt,IND,10%,SR10_5MA_10PER_1P35
Model_355 3-STATE,1.35V,ODT off,fast, 0.88*RExt,IND,10%,SR10_9MA_10PER_1P35
Model_356 3-STATE,1.35V,ODT off,slow, 1.60*RExt,IND,10%,SR01_5MA_10PER_1P35
Model_357 3-STATE,1.35V,ODT off,slowest, 1.60*RExt,IND,10%,SR11_5MA_10PER_1P35
Model_358 3-STATE,1.35V,ODT off,fastest, 1.14*RExt,IND,10%,SR00_7MA_10PER_1P35
Model_359 3-STATE,1.35V,ODT off,slow, 0.88*RExt,IND,10%,SR01_9MA_10PER_1P35
Model_360 3-STATE,1.35V,ODT off,fastest, 0.73*RExt,IND,10%,SR00_11MA_10PER_1P35
Model_361 3-STATE,1.35V,ODT off,fastest, 0.80*RExt,IND,10%,SR00_10MA_10PER_1P35
Model_362 3-STATE,1.35V,ODT off,fast, 0.73*RExt,IND,10%,SR10_11MA_10PER_1P35
Model_363 3-STATE,1.35V,ODT off,slowest, 1.14*RExt,IND,10%,SR11_7MA_10PER_1P35
Model_364 3-STATE,1.35V,ODT off,fast, 1.00*RExt,IND,10%,SR10_8MA_10PER_1P35
Model_365 3-STATE,1.35V,ODT off,slow, 0.73*RExt,IND,10%,SR01_11MA_10PER_1P35
Model_366 3-STATE,1.35V,ODT off,slow, 1.00*RExt,IND,10%,SR01_8MA_10PER_1P35
Model_367 3-STATE,1.35V,ODT off,fast, 0.67*RExt,IND,10%,SR10_12MA_10PER_1P35
Model_368 3-STATE,1.35V,ODT off,slowest, 1.00*RExt,IND,10%,SR11_8MA_10PER_1P35
Model_369 3-STATE,1.35V,ODT off,slow, 0.67*RExt,IND,10%,SR01_12MA_10PER_1P35
Model_370 3-STATE,1.35V,ODT off,fastest, 1.60*RExt,IND,10%,SR00_5MA_10PER_1P35
Model_371 3-STATE,1.35V,ODT off,fastest, 0.88*RExt,IND,10%,SR00_9MA_10PER_1P35
Model_372 3-STATE,1.35V,ODT off,fastest, 1.33*RExt,IND,10%,SR00_6MA_10PER_1P35
Model_373 3-STATE,1.35V,ODT off,fast, 1.14*RExt,IND,10%,SR10_7MA_10PER_1P35
Model_374 3-STATE,1.35V,ODT off,fast, 1.33*RExt,IND,10%,SR10_6MA_10PER_1P35
Model_375 3-STATE,1.35V,ODT off,slow, 1.14*RExt,IND,10%,SR01_7MA_10PER_1P35
Model_376 3-STATE,1.35V,ODT off,slowest, 0.88*RExt,IND,10%,SR11_9MA_10PER_1P35
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| Models and submodels in the file (1040): Model_1 (I/O), Model_2 (I/O), Model_3 (I/O), Model_4 (I/O), Model_5 (I/O), Model_6 (I/O), Model_7 (I/O), Model_8 (I/O), Model_9 (I/O), Model_10 (I/O), Model_11 (I/O), Model_12 (I/O), Model_13 (I/O), Model_14 (I/O), Model_15 (I/O), Model_16 (I/O), Model_17 (I/O), Model_18 (I/O), Model_19 (I/O), Model_20 (I/O), Model_21 (I/O), Model_22 (I/O), Model_23 (I/O), Model_24 (I/O), Model_25 (I/O), Model_26 (I/O), Model_27 (I/O), Model_28 (I/O), Model_29 (I/O), Model_30 (I/O), Model_31 (I/O), Model_32 (I/O), Model_33 (I/O), Model_34 (I/O), Model_35 (I/O), Model_36 (I/O), Model_37 (I/O), Model_38 (I/O), Model_39 (I/O), Model_40 (I/O), Model_41 (I/O), Model_42 (I/O), Model_43 (I/O), Model_44 (I/O), Model_45 (I/O), Model_46 (I/O), Model_47 (I/O), Model_48 (I/O), Model_49 (3-state), Model_50 (3-state), Model_51 (3-state), Model_52 (3-state), Model_53 (3-state), Model_54 (3-state), Model_55 (3-state), Model_56 (3-state), Model_57 (3-state), Model_58 (3-state), Model_59 (3-state), Model_60 (3-state), Model_61 (3-state), Model_62 (3-state), Model_63 (3-state), Model_64 (3-state), Model_65 (3-state), Model_66 (3-state), Model_67 (3-state), Model_68 (3-state), Model_69 (3-state), Model_70 (3-state), Model_71 (3-state), Model_72 (3-state), Model_73 (3-state), Model_74 (3-state), Model_75 (3-state), Model_76 (3-state), Model_77 (3-state), Model_78 (3-state), Model_79 (3-state), Model_80 (3-state)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
